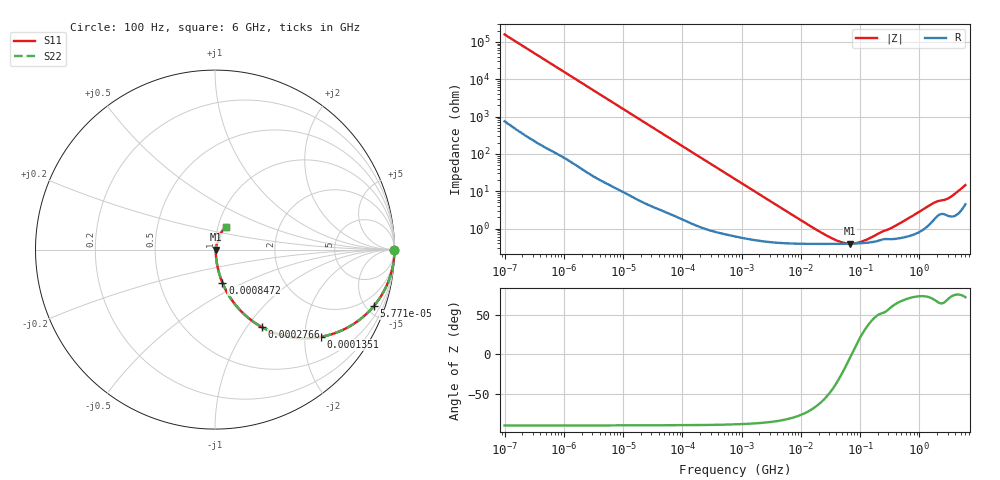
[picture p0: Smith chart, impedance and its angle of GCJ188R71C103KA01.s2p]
!Murata Part Number: GCJ188R71C103KA01
!These Parameters are Measured in Series Mode Connection
!Data Generated on Mar 13, 2026
!  o--ll--o
!Port1  Port2
!  o------o
!Operation Temp=25[degC], DC Bias Voltage=0[V]
!Freq. Start=100[Hz] Stop=6[GHz] 401[Steps]
# Hz S RI R 50
!Freq.(Hz) S11(Real) S11(Imag) S21(Real) S21(Imag) S12(Real) S12(Imag) S22(Real) S22(Imag)
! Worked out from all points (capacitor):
!   401 points, 100 Hz to 6 GHz, reference 50 ohm
!   read as one part in series: C = 10.1 nF near 109 Hz
!   lowest |Z| = 396 mohm at 68.17 MHz (marker M1)
!   series resonance near 71.67 MHz, so ESL is about 490 pH
!   S11 on the Smith chart (normalised r, x): 100 Hz: open; 57.71 kHz: 1.05, -5.58; 135.1 kHz: 1.03, -2.40; 276.6 kHz: 1.02, -1.17; 847.2 kHz: 1.01, -0.39; 6 GHz: 1.09, +0.28
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100  1 -0.000634  3.4e-06 0.000634  3.4e-06 0.000634  1 -0.000634
2008  0.9998 -0.0126  0.000221 0.0126  0.000221 0.0126  0.9998 -0.0126
12041  0.9939 -0.0747  0.00608 0.0747  0.00608 0.0747  0.9939 -0.0747
40335  0.9391 -0.2351  0.0609 0.2351  0.0609 0.2351  0.9391 -0.2351
57709  0.884 -0.3156  0.116 0.3156  0.116 0.3156  0.884 -0.3156
86348  0.7752 -0.4122  0.2248 0.4122  0.2248 0.4122  0.7752 -0.4122
135116  0.5884 -0.4863  0.4116 0.4863  0.4116 0.4863  0.5884 -0.4863
193316  0.4143 -0.486  0.5857 0.486  0.5857 0.486  0.4143 -0.486
276587  0.2599 -0.4308  0.7401 0.4308  0.7401 0.4308  0.2599 -0.4308
452617  0.1198 -0.3145  0.8802 0.3145  0.8802 0.3145  0.1198 -0.3145
774597  0.048 -0.1998  0.952 0.1998  0.952 0.1998  0.048 -0.1998
847162  0.0413 -0.1841  0.9587 0.1841  0.9587 0.1841  0.0413 -0.1841
2713602  0.00804 -0.0601  0.992 0.0601  0.992 0.0601  0.00804 -0.0601
1.555665e7  0.00398 -0.0101  0.996 0.0101  0.996 0.0101  0.00398 -0.0101
3.80911e7  0.00389 -0.0031  0.9961 0.0031  0.9961 0.0031  0.00389 -0.0031
5.211241e7  0.0039 -0.00149  0.9961 0.00149  0.9961 0.00149  0.0039 -0.00149
6.817316e7  0.00393 -0.000229  0.9961 0.000229  0.9961 0.000229  0.00393 -0.000229
1.115611e8  0.00408 0.00209  0.9959 -0.00209  0.9959 -0.00209  0.00408 0.00209
3.124326e8  0.00525 0.00818  0.9948 -0.00818  0.9948 -0.00818  0.00525 0.00818
1.712697e9  0.0181 0.0434  0.9819 -0.0434  0.9819 -0.0434  0.0181 0.0434
3.065283e9  0.0249 0.0575  0.9751 -0.0575  0.9751 -0.0575  0.0249 0.0575
6e9  0.0596 0.1254  0.9404 -0.1254  0.9404 -0.1254  0.0596 0.1254
